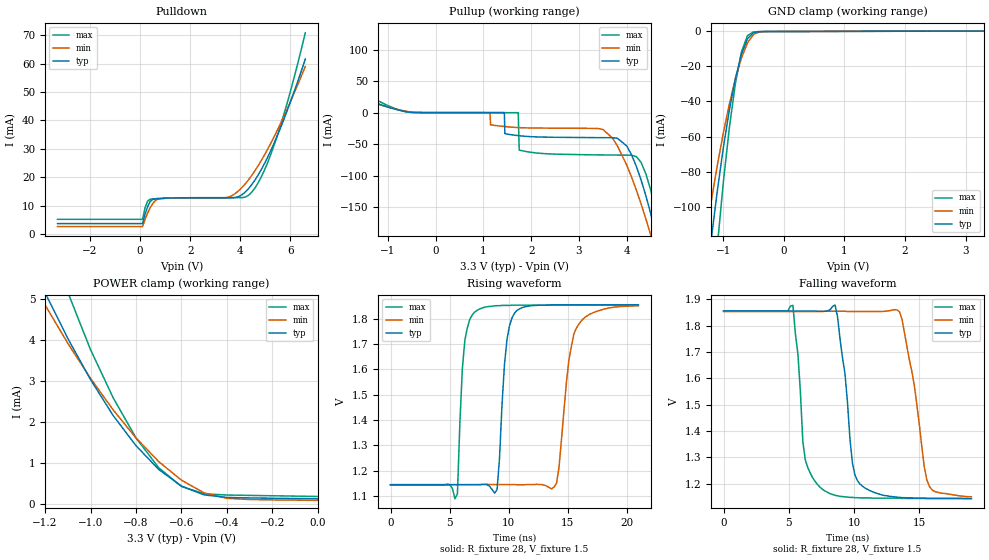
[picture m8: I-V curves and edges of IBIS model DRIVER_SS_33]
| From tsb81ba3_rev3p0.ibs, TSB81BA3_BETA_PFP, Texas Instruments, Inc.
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|   Model DRIVER_SS_33
[Model]   DRIVER_SS_33
Model_type   3-state
Polarity   Non-Inverting
Vmeas = 1.5V
Cref  = 10pF
Rref  = 28
Vref  = 1.5V
C_comp   7.16pF   4.20pF   8.10pF
|c_comp values are assumed by QualiM
[Temperature Range]   40   125   -40
[Voltage Range]   3.3V   3.0V   3.6V
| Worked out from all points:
|   slope of the pulldown table from 0 to 0.495 V, typ, clamps not added: 58.6 ohm
|   slope of the pullup table from 0 to 0.495 V, typ, clamps not added: 14.3 kohm
|   GND clamp passes 1 mA (typ) near -0.51 V on its own axis
|   POWER clamp passes 1 mA (typ) near -0.73 V on its own axis
|   rising waveform, R_fixture 28, V_fixture 1.5: 20-80 % time 583ps typ, 995ps min, 493ps max; typ from 1.14 V to 1.85 V
|   falling waveform, R_fixture 28, V_fixture 1.5: 20-80 % time 840ps typ, 1.23ns min, 645ps max; typ from 1.86 V to 1.14 V
[Pulldown]
| voltage   I(typ)   I(min)   I(max)
-3.3V     3.757mA    2.698mA    5.258mA
100mV     3.757mA    2.698mA    5.258mA
300mV     9.667mA    7.432mA    11.67mA
500mV     12.25mA    10.71mA    12.42mA
800mV     12.59mA    12.5mA     12.59mA
3.5V      12.84mA    12.95mA    12.86mA
3.9V      13.12mA    15.01mA    12.88mA
4.3V      15.72mA    18.77mA    13.52mA
4.8V      22.07mA    25.28mA    19.43mA
5.3V      30.93mA    33.32mA    29.96mA
5.9V      43.97mA    44.48mA    46.86mA
6.6V      61.57mA    58.96mA    70.81mA
[Pullup]
| voltage   I(typ)   I(min)   I(max)
-3.3V     92.43mA    71.65mA    134.8mA
-900mV    6.738mA    7.114mA    8.201mA
1.44V     50.14uA    -21.99mA   88.41uA
1.45V     -33.06mA   -22.06mA   87.54uA
1.73V     -36.45mA   -23.64mA   63.21uA
1.75V     -36.62mA   -23.71mA   -59.08mA
3.5V      -39.7mA    -26.6mA    -67.16mA
4V        -52.96mA   -83.64mA   -67.45mA
4.3V      -107.2mA   -145.3mA   -79.19mA
4.5V      -160.2mA   -194.3mA   -123.1mA
4.7V      -223.6mA   -248.5mA   -191.9mA
6.6V      -1.087A    -892.6mA   -1.38A
[GND_clamp]
| voltage   I(typ)   I(min)   I(max)
-3.3V     -1.046A    -757.5mA   -1.535A
-1.3V     -149.5mA   -119.5mA   -210.5mA
-1.2V     -119mA     -97.3mA    -164.7mA
-1.1V     -91.45mA   -76.81mA   -123.2mA
-1V       -66.62mA   -58.16mA   -86.45mA
-900mV    -44.99mA   -41.51mA   -55.05mA
-800mV    -26.96mA   -27.07mA   -29.75mA
-700mV    -13.08mA   -15.22mA   -11.74mA
-600mV    -4.253mA   -6.604mA   -2.443mA
-500mV    -783.8uA   -1.767mA   -330.8uA
-300mV    -129.9uA   -130.5uA   -158.4uA
3.3V      125.8uA    108.3uA    156.4uA
[POWER_clamp]
| voltage   I(typ)   I(min)   I(max)
-3.3V     43.1mA     35mA       61.9mA
-1.3V     6.366mA    5.851mA    8.441mA
-1.2V     5.148mA    4.849mA    6.721mA
-1.1V     4.035mA    3.917mA    5.16mA
-1V       3.033mA    3.062mA    3.763mA
-900mV    2.153mA    2.291mA    2.585mA
-800mV    1.423mA    1.611mA    1.613mA
-700mV    842.6uA    1.033mA    884.4uA
-600mV    436.4uA    581.1uA    427.7uA
-500mV    221.3uA    269.8uA    247.7uA
-400mV    159.4uA    138.1uA    218uA
0V        125.8uA    87.93uA    182.5uA
[Ramp]
| variable   typ   min   max
dV/dt_r 0.4266V/0.582714ns  0.4242V/0.995135ns  0.4266V/0.492663ns
dV/dt_f 0.4278V/0.839786ns  0.4224V/1.23378ns  0.4266V/0.645057ns
R_load = 28
[Rising Waveform]
R_fixture = 28
V_fixture = 1.5
V_fixture_min = 1.5
V_fixture_max = 1.5
| time   V(typ)   V(min)   V(max)
0s        1.144V     1.145V     1.144V
5.46ns    1.144V     1.145V     1.089V
5.67ns    1.144V     1.145V     1.108V
6.09ns    1.144V     1.145V     1.604V
6.51ns    1.144V     1.145V     1.764V
8.82ns    1.111V     1.145V     1.851V
10.08ns   1.772V     1.145V     1.853V
13.86ns   1.855V     1.135V     1.855V
15.75ns   1.855V     1.763V     1.855V
21ns      1.855V     1.852V     1.855V
[Falling Waveform]
R_fixture = 28
V_fixture = 1.5
V_fixture_min = 1.5
V_fixture_max = 1.5
| time   V(typ)   V(min)   V(max)
0s        1.856V     1.854V     1.855V
5.32ns    1.856V     1.854V     1.877V
6.27ns    1.856V     1.854V     1.29V
8.55ns    1.879V     1.855V     1.156V
9.31ns    1.618V     1.855V     1.15V
9.69ns    1.371V     1.854V     1.148V
10.07ns   1.234V     1.854V     1.147V
13.49ns   1.148V     1.853V     1.145V
15.77ns   1.144V     1.191V     1.144V
19ns      1.143V     1.15V      1.144V
